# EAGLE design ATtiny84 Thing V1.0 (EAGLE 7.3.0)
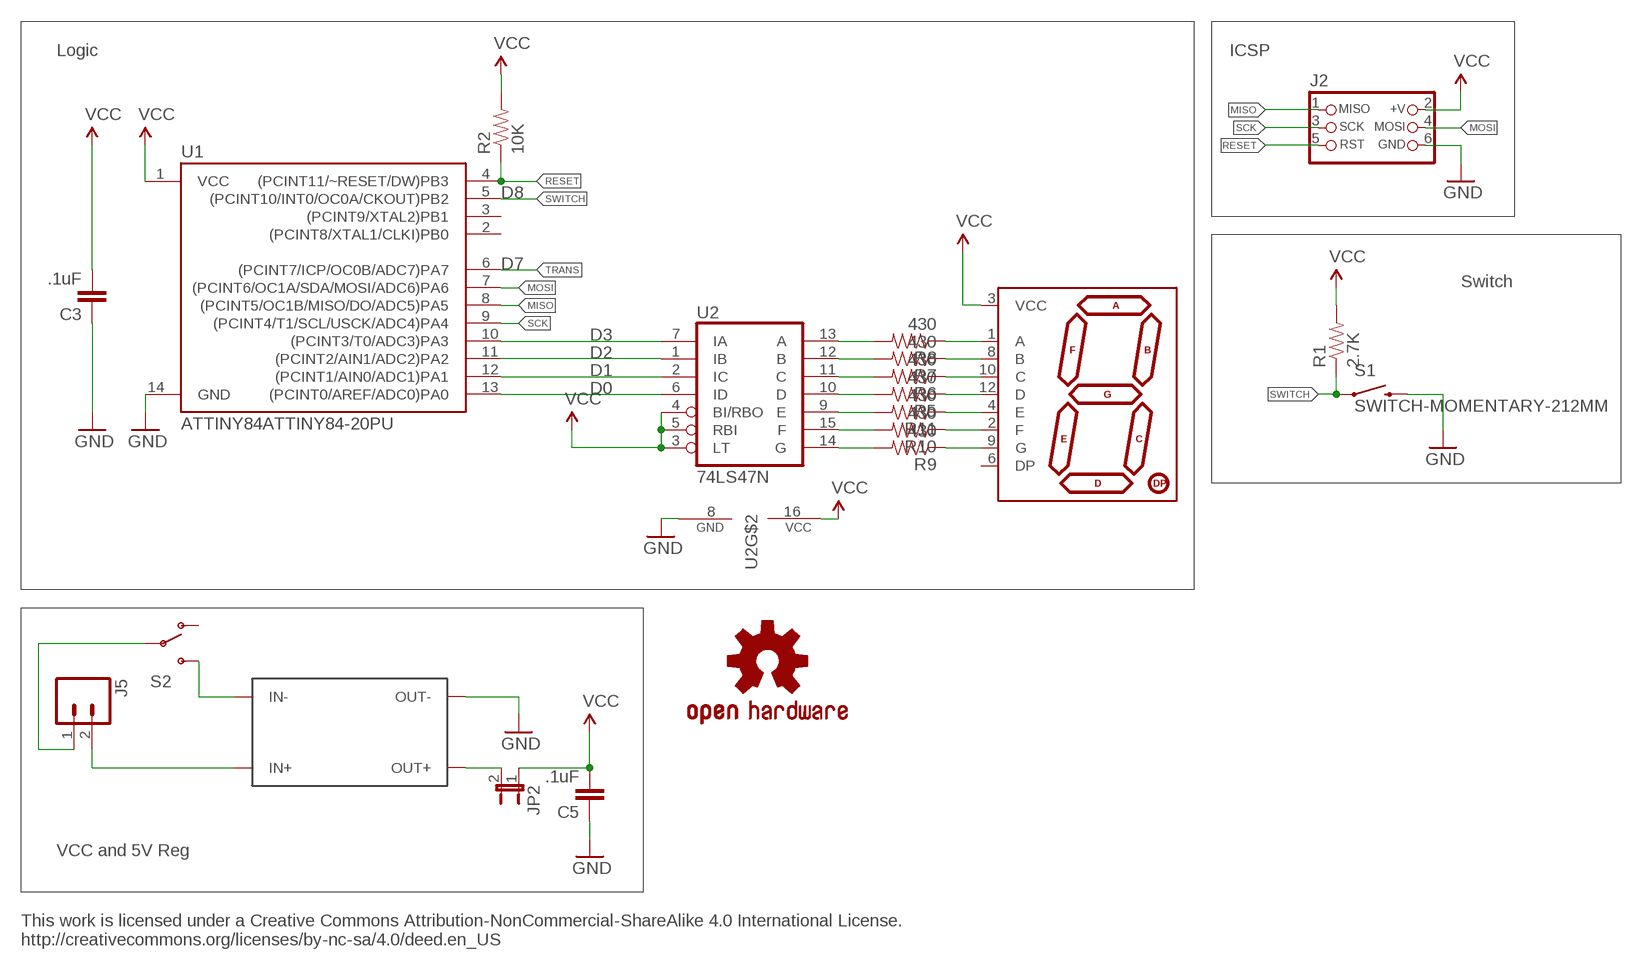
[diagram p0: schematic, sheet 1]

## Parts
C3  .1uF  CAP0805  [0805]
C5  .1uF  CAP0805  [0805]
J2  CON_HEADER_PRG_AVR_ICSP-PTH  [HEADER_PRG_2X03]
J5  M02JST-PTH-2  [JST-2-PTH]
JP2  JUMPER-2SMD-NO-NS  [SJ_2S-NO-NS]
LOGO1  OSHW-LOGOS  [OSHW-LOGO-S]
R1  2.7K  RESISTOR0805-RES  [0805]
R2  10K  RESISTOR0805-RES  [0805]
R5  430  RESISTOR0805-RES  [0805]
R6  430  RESISTOR0805-RES  [0805]
R7  430  RESISTOR0805-RES  [0805]
R8  430  RESISTOR0805-RES  [0805]
R9  430  RESISTOR0805-RES  [0805]
R10  430  RESISTOR0805-RES  [0805]
R11  430  RESISTOR0805-RES  [0805]
S1  SWITCH-MOMENTARY-212MM  [TACTILE-PTH-12MM]
S2  SWITCH-SPDT-SMD-A  [SWITCH-SPST-SMD-A]
U1  ATTINY84ATTINY84-20PU  [DIL14]
U2  74LS47N  [DIL16]
U$1  7-SEGMENT_HDSP-N150  [HDSP-N150]
U$3  DCTODC  [DCTODC]

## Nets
GND: C3.1 C5.1 J2.6(GND) S1.3 U1.14(GND) U2.8(GND) U$3.OUT-
MISO: J2.1(MISO) U1.8((PCINT5/OC1B/MISO/DO/ADC5)PA5)
MOSI: J2.4(MOSI) U1.7((PCINT6/OC1A/SDA/MOSI/ADC6)PA6)
N$3: U1.10((PCINT3/T0/ADC3)PA3) U2.7(IA)
N$4: U1.11((PCINT2/AIN1/ADC2)PA2) U2.1(IB)
N$5: R8.1 U$1.1(A)
N$6: R7.1 U$1.8(B)
N$7: R6.2 U2.11(C)
N$8: R5.2 U2.10(D)
N$9: R11.2 U2.9(E)
N$10: R10.2 U2.15(F)
N$11: R9.1 U$1.9(G)
N$12: R8.2 U2.13(A)
N$13: R7.2 U2.12(B)
N$14: R10.1 U$1.2(F)
N$15: R11.1 U$1.4(E)
N$16: R5.1 U$1.12(D)
N$17: R6.1 U$1.10(C)
N$18: R9.2 U2.14(G)
N$19: U1.12((PCINT1/AIN0/ADC1)PA1) U2.2(IC)
N$20: U1.13((PCINT0/AREF/ADC0)PA0) U2.6(ID)
N$21: J5.1 S2.2(P)
N$23: J5.2 U$3.IN+
N$27: JP2.2 U$3.OUT+
N$28: S2.3(S) U$3.IN-
RESET: J2.5(RST) R2.1 U1.4((PCINT11/~RESET/DW)PB3)
SCK: J2.3(SCK) U1.9((PCINT4/T1/SCL/USCK/ADC4)PA4)
SWITCH: R1.1 S1.1 U1.5((PCINT10/INT0/OC0A/CKOUT)PB2)
TRANS: U1.6((PCINT7/ICP/OC0B/ADC7)PA7)
VCC: C3.2 C5.2 J2.2(+V) JP2.1 R1.2 R2.2 U1.1(VCC) U2.3(LT) U2.4(BI/RBO) U2.5(RBI) U2.16(VCC) U$1.3(VCC)
Unconnected: S2.1(O) U1.2((PCINT8/XTAL1/CLKI)PB0) U1.3((PCINT9/XTAL2)PB1) U$1.6(DP)

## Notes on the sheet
- Logic | ICSP
- D8
- D7
- Switch
- D3
- D2
- D1
- D0
- VCC and 5V Reg
- This work is licensed under a Creative Commons Attribution-NonCommercial-ShareAlike 4.0 International License.
  http://creativecommons.org/licenses/by-nc-sa/4.0/deed.en_US

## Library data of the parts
C3 C5 = SparkFun-Capacitors:CAP: Capacitor
J2 = dp_devices:CON_HEADER_PRG_AVR_ICSP: 2x3 AVR ICSP programming header
J5 = SparkFun-Connectors:M02: Standard 2-pin 0.1" header. Use with; PROD_ID: CONN-09863; SKU: PRT-09914
JP2 = SparkFun-Retired:JUMPER-2: Jumper
LOGO1 = SparkFun-Aesthetics:OSHW-LOGO: Open Source Hardware Logo
R1 R2 R5-R11 = SparkFun-Resistors:RESISTOR: Resistor
S1 = SparkFun-Electromechanical:SWITCH-MOMENTARY-2: Various NO switches- pushbuttons, reed, etc; PROD_ID: SWCH-09185
S2 = SparkFun-Electromechanical:SWITCH-SPDT: SPDT Switch Simple slide switch, Spark Fun Electronics SKU : COM-00102 DPDT SMT slide switch, AYZ0202, SWCH-08179; PROD_ID: SWCH-10651
U1 = SparkFun-DigitalIC:ATTINY84: Atmel 14-pin 2/4/8kB flash uC
U2 = 74xx-us:74*47: BCD to seven segment DECODER/DRIVER Source: http://www.ee.washington.edu/stores/DataSheets/74ls/74ls47.pdf
U$1 = 7-Segment HDSP-N150:7-SEGMENT_HDSP-N150
U$3 = DC to DC:DCTODC

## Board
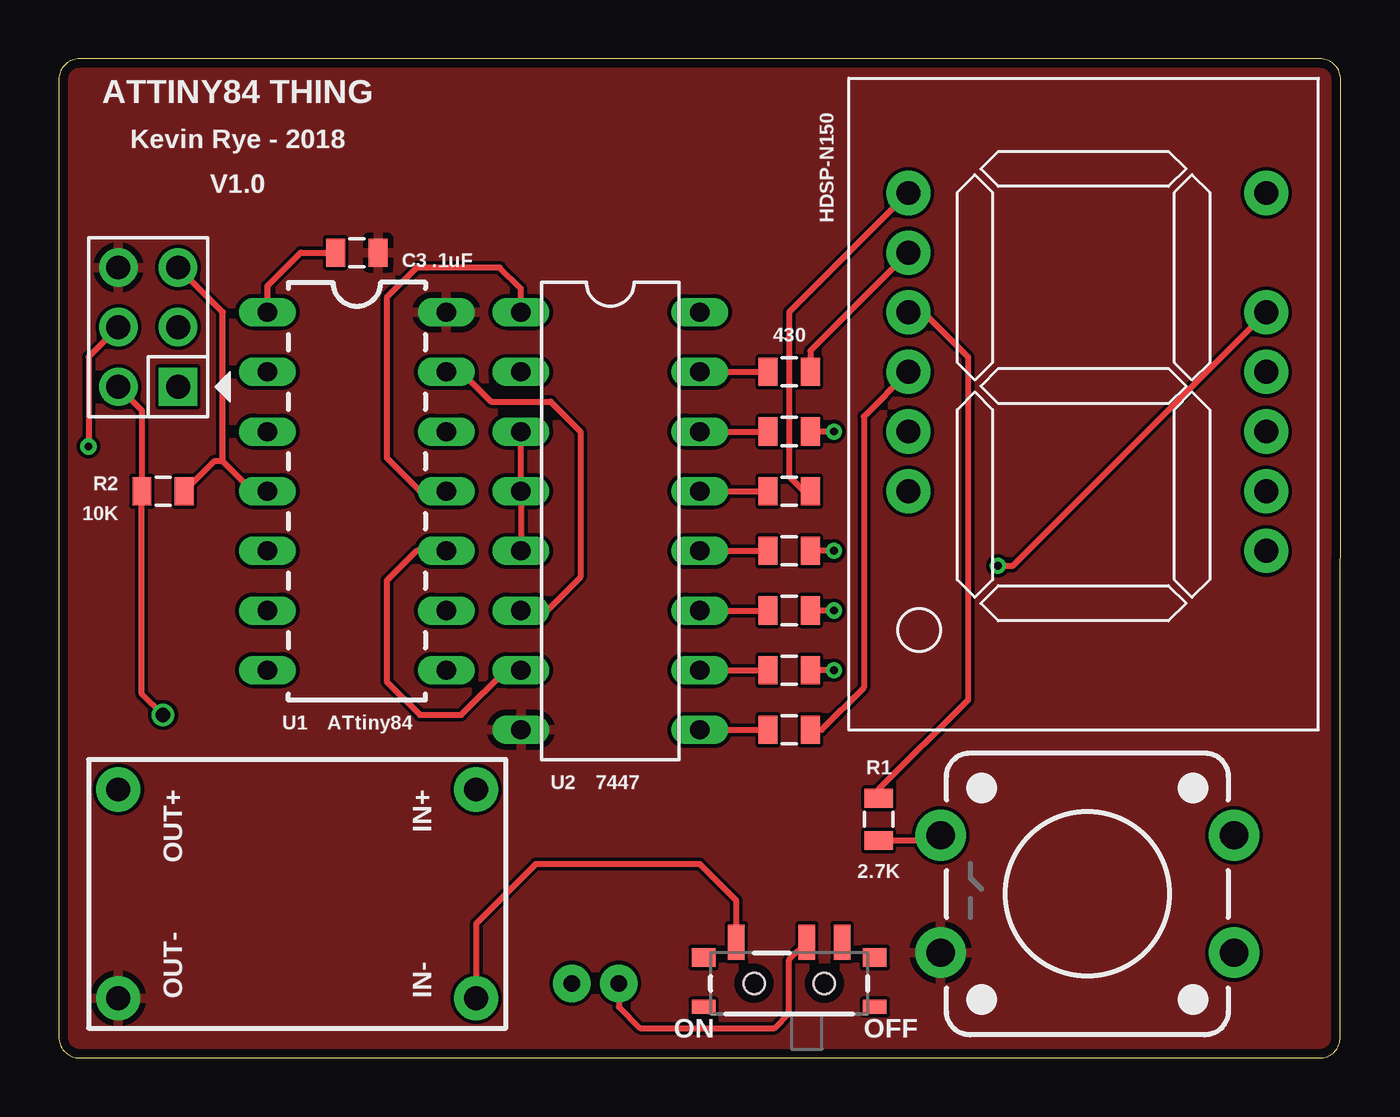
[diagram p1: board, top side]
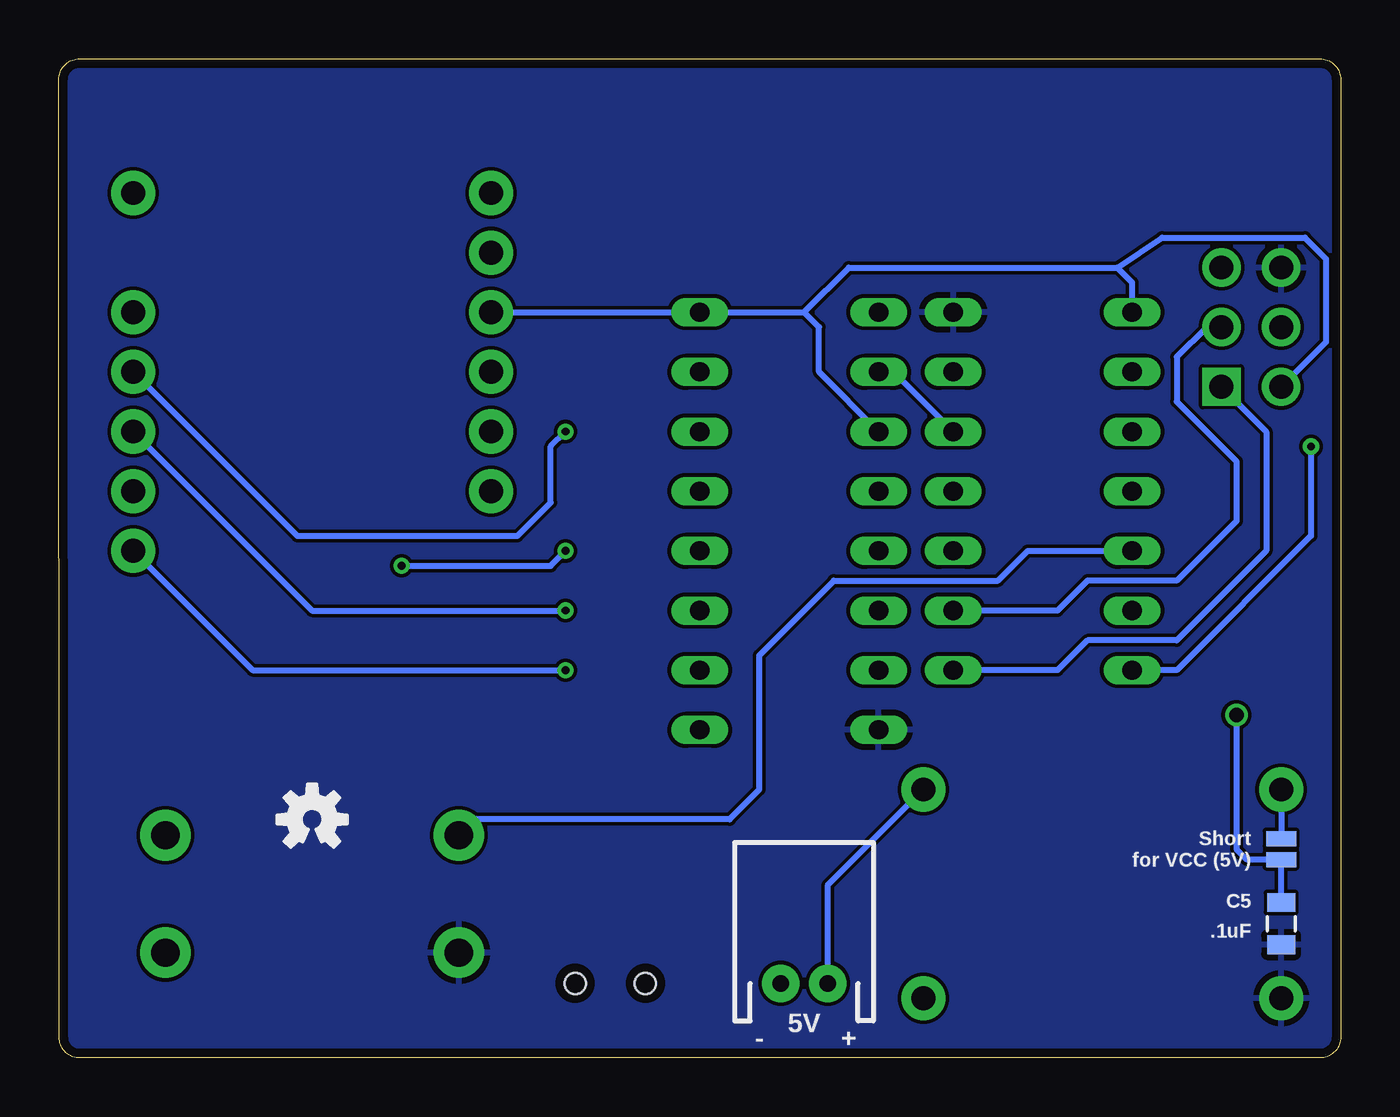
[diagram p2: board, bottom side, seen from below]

Size 54.61 x 42.55 mm. Coordinates in mm from the lower left corner, seen from the top.
Outline: 0,41.65 0,0.9 arc90 0.9,0 53.71,0 arc90 54.59,0.88 54.61,41.65 arc90 53.71,42.55 0.9,42.55 arc90 0,41.65
Copper layers (1*16): Top 0.0356mm / dielectric 1.5011mm / Bottom 0.0356mm
Design rules "oshpark-2layer": minimum track width 6mil, minimum drill 13mil, track to track 6mil, track to pad 6mil, pad to pad 6mil, via to via 6mil, smd to smd 6mil, copper to edge 15mil, drill to drill 6mil, minimum pad ring 7mil, minimum via ring 7mil, stop-mask expansion 2.5mil, vias tented up to drill 0mil, thermal gap 10mil

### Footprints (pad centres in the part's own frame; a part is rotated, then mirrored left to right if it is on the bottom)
0805 = smd 0.8 x 1.2: 1 -0.9,0; 2 0.9,0
HEADER_PRG_2X03 = drill 1.02 pad 1.632 square: 1 -2.54,-1.27 | drill 1.02 pad 1.632: 2 -2.54,1.27; 3 0,-1.27; 4 0,1.27; 5 2.54,-1.27; 6 2.54,1.27
JST-2-PTH = drill 0.7 pad 1.6: 1 -1,0; 2 1,0
SJ_2S-NO-NS = smd 0.635 x 1.27: 1 -0.45,0; 2 0.45,0
TACTILE-PTH-12MM = drill 1.2 pad 2.159: 1 6.25,-2.5; 2 -6.25,-2.5; 3 6.25,2.5; 4 -6.25,2.5
SWITCH-SPST-SMD-A = smd 0.7 x 1.5: 1 -2.25,-1.75; 2 -0.75,-1.75; 3 2.25,-1.75 | smd 1 x 0.6: GND1 -3.65,1; GND3 3.65,1 | smd 1 x 0.8: GND2 -3.65,-1.1; GND4 3.65,-1.1 | hole 0.9: -1.5,0; 1.5,0
DIL14 = drill 0.813 long: 1 -8.89,-3.81; 2 -6.35,-3.81; 3 -3.81,-3.81; 4 -1.27,-3.81; 5 1.27,-3.81; 6 3.81,-3.81; 7 6.35,-3.81; 8 6.35,3.81; 9 3.81,3.81; 10 1.27,3.81; 11 -1.27,3.81; 12 -3.81,3.81; 13 -6.35,3.81; 14 -8.89,3.81
DIL16 = drill 0.813 long: 1 -8.89,-3.81; 2 -6.35,-3.81; 3 -3.81,-3.81; 4 -1.27,-3.81; 5 1.27,-3.81; 6 3.81,-3.81; 7 6.35,-3.81; 8 8.89,-3.81; 9 8.89,3.81; 10 6.35,3.81; 11 3.81,3.81; 12 1.27,3.81; 13 -1.27,3.81; 14 -3.81,3.81; 15 -6.35,3.81; 16 -8.89,3.81
HDSP-N150 = drill 1.016 pad 1.88: 1 2.54,22.86; 2 2.54,20.32; 3 2.54,17.78; 4 2.54,15.24; 5 2.54,12.7; 6 2.54,10.16; 7 17.78,22.86; 8 17.78,17.78; 9 17.78,15.24; 10 17.78,12.7; 11 17.78,10.16; 12 17.78,7.62
DCTODC = drill 1.016 pad 1.88: IN+ 10.16,1.27; IN- 1.27,1.27; OUT+ 10.16,16.51; OUT- 1.27,16.51

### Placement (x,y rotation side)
C3  12.7,34.29 180 top
C5  2.54,5.71 90 bottom
J2  3.81,31.11 90 top
J5  22.86,3.17 0 bottom
JP2  2.54,8.89 90 bottom
LOGO1  43.81,10.16 0 bottom
R1  34.92,10.16 90 top
R2  4.45,24.13 180 top
R5  31.11,16.51 180 top
R6  31.11,19.05 180 top
R7  31.11,21.59 180 top
R8  31.11,24.13 180 top
R9  31.11,26.67 180 top
R10  31.11,29.21 180 top
R11  31.11,13.97 180 top
S1  43.81,6.99 180 top
S2  31.11,3.17 180 top
U1  12.7,22.86 270 top
U2  23.5,22.86 270 top
U$1  33.66,13.97 0 top
U$3  19.05,1.27 90 top

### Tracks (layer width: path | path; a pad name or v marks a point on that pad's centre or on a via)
GND
  pour Bottom: -0.64,43.18 55.24,43.18 55.24,-0.64 -0.64,-0.64
  pour Top: -1.27,43.81 55.88,43.81 55.88,-1.27 -1.27,-1.27
MISO
  Bottom 0.254: U1.8 12.06,16.51 10.79,17.78 6.99,17.78 3.17,21.59 3.17,26.67 J2.1
MOSI  (via drill 0.33)
  Top 0.254: v1.27,26.04 1.27,29.84 J2.4
  Bottom 0.254: U1.7 6.99,16.51 1.27,22.23 v1.27,26.04
N$3
  Top 0.254: U2.7 19.05,16.51 17.14,14.61 15.39,14.61 13.97,16.02 13.97,20.32 15.24,21.59 U1.10
N$4
  Top 0.254: U1.11 15.39,24.13 13.97,25.55 13.97,32.38 15.24,33.66 18.79,33.66 19.68,32.76 U2.1
N$5
  Top 0.254: R8.1 31.75,24.13 31.11,24.77 31.11,31.75 U$1.1
N$6  (via drill 0.33)
  Top 0.254: v33.02,21.59 R7.1 | v40.01,20.95 40.64,20.95 U$1.8
  Bottom 0.254: v33.02,21.59 33.66,20.95 v40.01,20.95
N$7
  Top 0.254: U2.11 R6.2
N$8
  Top 0.254: U2.10 R5.2
N$9
  Top 0.254: U2.9 R11.2
N$10
  Top 0.254: U2.15 R10.2
N$11  (via drill 0.33)
  Top 0.254: v33.02,26.67 R9.1
  Bottom 0.254: v33.02,26.67 33.66,26.04 33.66,23.64 35.08,22.23 44.45,22.23 U$1.9
N$12
  Top 0.254: U2.13 R8.2
N$13
  Top 0.254: U2.12 R7.2
N$14
  Top 0.254: U$1.2 32.02,30.11 R10.1
N$15
  Top 0.254: R11.1 32.49,13.97 34.29,15.77 34.29,27.3 U$1.4
N$16  (via drill 0.33)
  Top 0.254: v33.02,16.51 R5.1
  Bottom 0.254: v33.02,16.51 46.35,16.51 U$1.12
N$17  (via drill 0.33)
  Top 0.254: v33.02,19.05 R6.1 31.75,19.05
  Bottom 0.254: v33.02,19.05 43.81,19.05 U$1.10
N$18
  Top 0.254: U2.14 R9.2
N$19
  Bottom 0.254: U1.12 19.05,29.21 U2.2
N$20
  Top 0.254: U2.6 20.8,19.05 22.23,20.47 22.23,26.67 20.95,27.94 18.41,27.94 17.14,29.21 U1.13
N$21
  Top 0.254: S2.2 31.11,4.17 31.11,1.91 30.48,1.27 24.77,1.27 23.86,2.17 J5.1
N$23
  Bottom 0.254: U$3.IN+ 21.86,7.35 J5.2
N$27
  Bottom 0.254: U$3.OUT+ JP2.2
N$28
  Top 0.254: S2.3 28.86,6.7 27.3,8.26 20.32,8.26 17.78,5.71 U$3.IN-
RESET
  Top 0.254: 6.99,25.4 8.26,24.13 U1.4 | J2.5 6.99,31.75 6.99,25.4 | 6.99,25.4 6.62,25.4 R2.1
SCK
  Bottom 0.254: U1.9 12.06,19.05 10.79,20.32 6.99,20.32 4.45,22.86 4.45,25.4 6.99,27.94 6.99,29.84 5.71,31.11 J2.3
SWITCH
  Top 0.254: R1.1 37.34,9.26 S1.1
  Bottom 0.254: U1.5 13.34,21.59 14.61,20.32 21.59,20.32 24.77,17.14 24.77,11.43 26.04,10.16 36.89,10.16 S1.1
VCC  (via drill 0.61)
  Top 0.254: U2.5 U2.4 U2.3 | U1.1 8.89,32.87 10.31,34.29 C3.2 | U$1.3 36.83,31.75 38.73,29.84 38.73,15.24 34.92,11.43 R1.2 | J2.2 3.54,27.57 R2.2 3.54,15.51 v4.45,14.61
  Bottom 0.254: U$1.3 U2.16 22.86,31.75 | 9.53,33.66 8.89,33.02 U1.1 | 9.53,33.66 20.95,33.66 22.86,31.75 | U2.3 22.23,29.21 22.23,31.11 22.86,31.75 | 9.53,33.66 7.62,34.92 1.53,34.92 0.64,34.03 0.64,30.48 J2.2 | C5.2 JP2.1 4,8.44 4.45,8.89 v4.45,14.61

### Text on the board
Unrouted: This work is licensed under a Creative Commons Attribution-NonCommercial-ShareAlike 4.0 International License. / http://creativecommons.org/licenses/by-nc-sa/4.0/deed.en_US
tNames: ATTINY84 THING | Kevin Rye - 2018 | V1.0 | HDSP-N150 | ATtiny84 | 7447 | ON | OFF
bNames: Short / for VCC (5V) | 5V | + | -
